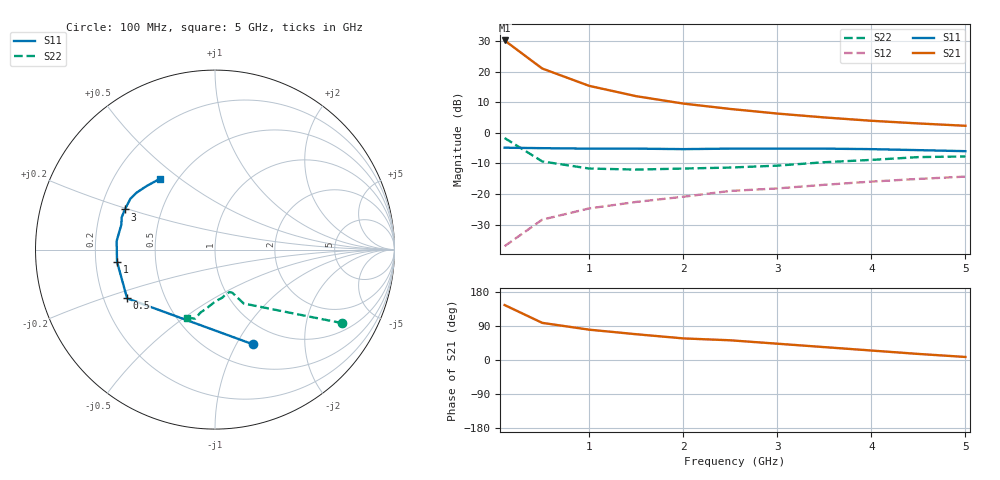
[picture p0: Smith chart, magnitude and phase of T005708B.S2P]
!AT-00570
!S-PARAMETERS at Vce=8V  Ic=20mA.  LAST UPDATED 07-21-92
!OBSOLETED Feb 1994 - nearest replacement: AT-41470
# ghz s ma r 50
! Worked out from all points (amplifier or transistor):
!   11 points, 100 MHz to 5 GHz, reference 50 ohm
!   highest |S21| = 30.2 dB at 100 MHz (marker M1)
!   |S21| within 3 dB of that: start of sweep to 230.8 MHz
!   unconditionally stable (mu >= 1): 1.034 GHz to end of sweep
!   at 500 MHz: K = 0.73, MSG = 24.7 dB, |S12| = -28.4 dB
!   at 2.5 GHz: K = 1.18, MAG = 10.8 dB, |S12| = -19.0 dB
!   at 5 GHz: K = 1.19, MAG = 5.7 dB, |S12| = -14.3 dB
!   S11 on the Smith chart (normalised r, x): 100 MHz: 0.75, -1.18; 500 MHz: 0.30, -0.24; 1 GHz: 0.29, -0.06; 3 GHz: 0.30, +0.19; 5 GHz: 0.40, +0.42
0.1  0.57 -68.0  32.27 145.0  0.014 64.0  0.82 -30.0
0.5  0.56 -151.0  11.22 98.0  0.038 47.0  0.34 -62.0
1  0.55 -173.0  5.84 80.0  0.058 53.0  0.26 -68.0
1.5  0.55 175.0  3.96 68.0  0.074 55.0  0.25 -71.0
2  0.54 165.0  3 57.0  0.09 52.0  0.26 -78.0
2.5  0.55 161.0  2.45 52.0  0.112 54.0  0.27 -81.0
3  0.55 156.0  2.06 43.0  0.123 51.0  0.29 -90.0
3.5  0.55 149.0  1.78 34.0  0.141 48.0  0.33 -98.0
4  0.54 144.0  1.57 25.0  0.159 43.0  0.36 -103.0
4.5  0.52 137.0  1.42 16.0  0.176 39.0  0.4 -106.0
5  0.5 128.0  1.3 8.0  0.192 35.0  0.41 -112.0
